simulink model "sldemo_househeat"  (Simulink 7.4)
settings: Solver=ode45  SolverMode=SingleTasking  StartTime=0.0  StopTime=48  FixedStep=1  RelTol=1e-3  AbsTol=1e-6
model workspace: external: M-Code (data not in the file)
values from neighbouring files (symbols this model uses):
  M = 1644.0 + 125.0    (= 1769)    [prb2.m]
undefined symbols (not defined in the file or in its folder): c, cost, Mdot, Req, THeater, TinIC
libraries: simulink_extras x3

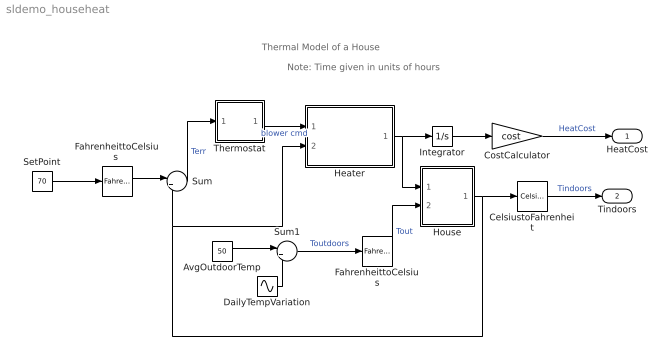
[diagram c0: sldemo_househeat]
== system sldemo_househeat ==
  note: Thermal Model of a House
  note: Note: Time given in units of hours
  AvgOutdoorTemp : Constant  Description=|  Value=50  OutDataType=sfix(16)  OutScaling=2^0
      | begin dimension                         
      | output _ : [(temperature fehrenheit 1)];
      | end dimension
  CelsiustoFahrenheit : simulink_extras/Transformations/Celsius to Fahrenheit  Description=|  SystemSampleTime=-1
      | begin dimension                        
      | input 1 : [(temperature fehrenheit 1)];
      | output 1 : [(temperature celsius 1)];  
      | end dimension
  CostCalculator : Gain  Description=|  Gain=cost  ParameterDataType=sfix(16)  ParameterScaling=2^0  OutDataType=sfix(16)  OutScaling=2^0
      | begin dimension                                                                    
      | constant _ : [(length metre -2, mass kilogram -1, time hour 2, currency dollar 1)];
      | end dimension
  DailyTempVariation : Sin  Description=|  Amplitude=15  Bias=0  Frequency=2*pi/24  Phase=0  Samples=10  SampleTime=0
      | begin dimension                         
      | output _ : [(temperature fehrenheit 1)];
      | end dimension
  FahrenheittoCelsius : simulink_extras/Transformations/Fahrenheit to Celsius  Description=|  SystemSampleTime=-1
      | begin dimension                        
      | input 1 : [(temperature fehrenheit 1)];
      | output 1 : [(temperature celsius 1)];  
      | end dimension
  "FahrenheittoCelsius " : simulink_extras/Transformations/Fahrenheit to Celsius  Description=|  SystemSampleTime=-1
      | begin dimension                        
      | input 1 : [(temperature fehrenheit 1)];
      | output 1 : [(temperature celsius 1)];  
      | end dimension
  Heater : Subsystem
  House : Subsystem
  Integrator : Integrator
  SetPoint : Constant  Description=|  Value=70  OutDataType=sfix(16)  OutScaling=2^0
      | begin dimension                         
      | output _ : [(temperature fehrenheit 1)];
      | end dimension
  Sum : Sum  Inputs=|+-  OutDataType=sfix(16)  OutScaling=2^0
  Sum1 : Sum  Inputs=|++  OutDataType=sfix(16)  OutScaling=2^0
  Thermostat : Subsystem
  HeatCost : Outport  Description=|  OutDataType=fixdt(1, 16)  OutScaling=2^0
      | begin dimension                 
      | input _ : [(currency dollar 1)];
      | end dimension
  Tindoors : Outport  Description=|  Port=2  OutDataType=fixdt(1, 16)  OutScaling=2^0
      | begin dimension                        
      | input _ : [(temperature fehrenheit 1)];
      | end dimension
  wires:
  Integrator/1 -> CostCalculator/1
  Thermostat/1(BlowerSwitch) -> Heater/1(OnOff)  "blower cmd"
  Sum/1 -> Thermostat/1(Terr)  "Terr"
  House/1(RoomTempTroom) -> CelsiustoFahrenheit/1, Sum/2, Heater/2(Troom)
  DailyTempVariation/1 -> Sum1/2
  Sum1/1 -> FahrenheittoCelsius/1  "Toutdoors"
  AvgOutdoorTemp/1 -> Sum1/1
  CelsiustoFahrenheit/1 -> Tindoors/1  "Tindoors"
  FahrenheittoCelsius/1 -> House/2(OutdoorTempTout)  "Tout"
  Heater/1(HeatFlow) -> Integrator/1, House/1(HeaterQDotIn)
  "FahrenheittoCelsius "/1 -> Sum/1
  SetPoint/1 -> "FahrenheittoCelsius "/1
  CostCalculator/1 -> HeatCost/1  "HeatCost"

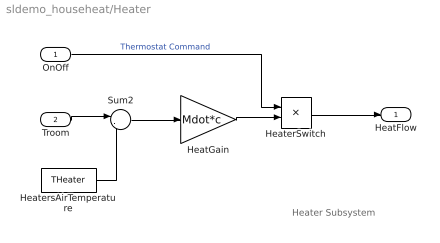
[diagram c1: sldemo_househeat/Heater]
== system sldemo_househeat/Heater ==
  note: Heater Subsystem
  OnOff : Inport  Description=|  OutDataType=sfix(16)  OutScaling=2^0
      | begin dimension       
      | output _ : [(dimensionless)];
      | end dimension
  Troom : Inport  Description=|  Port=2  OutDataType=sfix(16)  OutScaling=2^0
      | begin dimension                      
      | output _ : [(temperature celsius 1)];
      | end dimension
  HeatGain : Gain  Description=|  Gain=Mdot*c  ParameterDataType=sfix(16)  ParameterScaling=2^0  OutDataType=sfix(16)  OutScaling=2^0
      | begin dimension                                                                        
      | constant _ : [(length metre 2, mass kilogram 1, time hour -3, temperature celsius -1)];
      | end dimension
  HeaterSwitch : Product  OutDataType=sfix(16)  OutScaling=2^0
  HeatersAirTemperature : Constant  Description=|  Value=THeater  OutDataType=sfix(16)  OutScaling=2^0
      | begin dimension                      
      | output _ : [(temperature celsius 1)];
      | end dimension
  Sum2 : Sum  Inputs=|-+  OutDataType=sfix(16)  OutScaling=2^0
  HeatFlow : Outport  Description=|  OutDataType=sfix(16)  OutScaling=2^0
      | begin dimension                                             
      | input _ : [(length metre 2, mass kilogram 1, time hour -3)];
      | end dimension
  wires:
  HeatersAirTemperature/1 -> Sum2/2
  Troom/1 -> Sum2/1
  Sum2/1 -> HeatGain/1
  OnOff/1 -> HeaterSwitch/1  "Thermostat Command"
  HeatGain/1 -> HeaterSwitch/2
  HeaterSwitch/1 -> HeatFlow/1

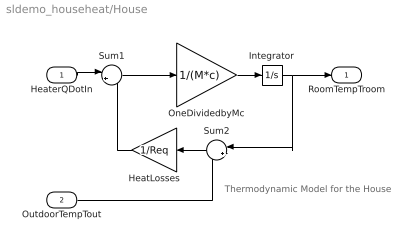
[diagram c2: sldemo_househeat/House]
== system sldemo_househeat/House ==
  note: Thermodynamic Model for the House
  HeaterQDotIn : Inport  Description=|  OutDataType=sfix(16)  OutScaling=2^0
      | begin dimension                                              
      | OUTPUT _ : [(length metre 2, mass kilogram 1, time hour -3)];
      | end dimension
  OutdoorTempTout : Inport  Description=|  Port=2  OutDataType=sfix(16)  OutScaling=2^0
      | begin dimension                      
      | output _ : [(temperature celsius 1)];
      | end dimension
  HeatLosses : Gain  Description=|  Gain=1/Req  ParameterDataType=sfix(16)  ParameterScaling=2^0  OutDataType=sfix(16)  OutScaling=2^0
      | begin dimension                                                                        
      | constant _ : [(length metre 2, mass kilogram 1, time hour -3, temperature celsius -1)];
      | end dimension
  Integrator : Integrator  InitialCondition=TinIC
  OneDividedbyMc : Gain  Description=|  Gain=1/(M*c)  ParameterDataType=sfix(16)  ParameterScaling=2^0  OutDataType=sfix(16)  OutScaling=2^0
      | begin dimension                                                                        
      | constant _ : [(length metre -2, mass kilogram -1, time hour 2, temperature celsius 1)];
      | end dimension
  Sum1 : Sum  Inputs=|+-  OutDataType=sfix(16)  OutScaling=2^0
  Sum2 : Sum  Inputs=|+-  OutDataType=sfix(16)  OutScaling=2^0
  RoomTempTroom : Outport  Description=|  OutDataType=sfix(16)  OutScaling=2^0  InitialOutput=0
      | begin dimension                     
      | input _ : [(temperature celsius 1)];
      | end dimension
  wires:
  OutdoorTempTout/1 -> Sum2/2
  HeaterQDotIn/1 -> Sum1/1
  Sum1/1 -> OneDividedbyMc/1
  Sum2/1 -> HeatLosses/1
  HeatLosses/1 -> Sum1/2
  OneDividedbyMc/1 -> Integrator/1
  Integrator/1 -> Sum2/1, RoomTempTroom/1

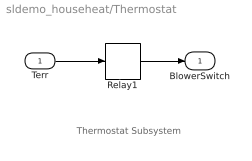
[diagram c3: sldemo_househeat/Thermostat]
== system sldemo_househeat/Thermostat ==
  note: Thermostat Subsystem
  Terr : Inport  Description=|  OutDataType=sfix(16)  OutScaling=2^0
      | begin dimension                      
      | output _ : [(temperature celsius 1)];
      | end dimension
  Relay1 : Relay  OnSwitchValue=5*(5/9)  OffSwitchValue=-5*(5/9)  OutDataType=sfix(16)  OutScaling=2^0
  BlowerSwitch : Outport  Description=|  OutDataType=sfix(16)  OutScaling=2^0  InitialOutput=0
      | begin dimension      
      | input _ : [(dimensionless)];
      | end dimension
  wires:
  Terr/1 -> Relay1/1
  Relay1/1 -> BlowerSwitch/1
